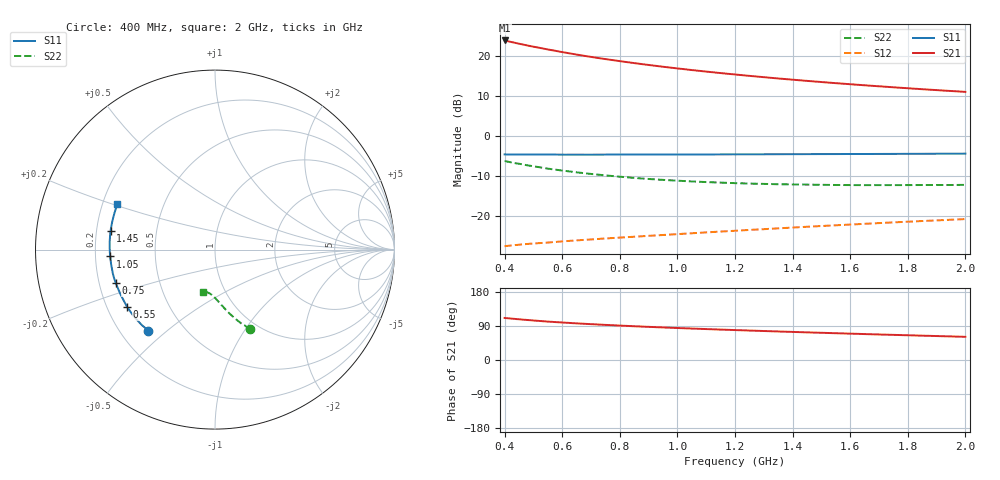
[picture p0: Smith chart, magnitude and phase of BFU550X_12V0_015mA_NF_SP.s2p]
! Filename:  P:\Prog\Test\Noise\ATS_data\Testdata_Net\BFU550X attenuator noise\BFU550X_APG2013_44_C05_12p0V_015mA_NF_CM01_D.sf
! Date/Time: Fri 26/Jul/2013 14:34:25
! BFU550X_APG2013_44_C05_12p0V_1to35mA_NF_CM01_Bias6_R.sf
! Noise Parameter Data File
! BFU550X_APG2013_44_C05_12p0V_1to35mA_NF_CM01
! Date/time: Mon Jul 22 11:28:10 2013
! VAR V_out= 12.001000
! VAR I_out= 14.995000
! VAR V_in= 0.783400
! VAR I_in= 0.144350
! Device data file deembeded for feedlines and parallel
! Original file: \BFU550X attenuator noise\BFU550X_APG2013_44_C05_12p0V_015mA_NF_CM01_R.sf
! Feed-files: PR005V01_100713_Feed1.s2p, PR005V01_100713_Feed2.s2p
! Parallel-file: PR005V01_100713_Par.s2p
# MHz S MA R 50
!  Freq-MHz  S11-mag  S11-arg  S21-mag  S21-arg  S12-mag  S12-arg  S22-mag  S22-arg
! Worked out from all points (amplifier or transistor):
!   37 points, 400 MHz to 2 GHz, reference 50 ohm
!   highest |S21| = 23.9 dB at 400 MHz (marker M1)
!   |S21| within 3 dB of that: start of sweep to 606.9 MHz
!   unconditionally stable (mu >= 1): 1.771 GHz to end of sweep
!   at 500 MHz: K = 0.51, MSG = 24.7 dB, |S12| = -27.0 dB
!   at 1.1 GHz: K = 0.85, MSG = 20.2 dB, |S12| = -24.2 dB
!   at 2 GHz: K = 1.03, MAG = 14.9 dB, |S12| = -20.8 dB
!   lowest NFmin = 0.94 dB at 460 MHz
!   S11 on the Smith chart (normalised r, x): 400 MHz: 0.31, -0.43; 550 MHz: 0.28, -0.28; 750 MHz: 0.27, -0.15; 1.05 GHz: 0.26, -0.03; 1.45 GHz: 0.26, +0.08; 2 GHz: 0.26, +0.21
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400  0.5867 -129.6  15.71 110.9  0.04152 44.7  0.4844 -66.1
420  0.5844 -132.1  15.11 109.5  0.04224 44.5  0.4679 -67.6
440  0.5854 -134.7  14.58 108.1  0.04297 44.1  0.4533 -68.7
460  0.5851 -137.1  14.06 106.8  0.04367 43.8  0.4418 -70.0
500  0.5853 -141.5  13.13 104.3  0.04487 43.4  0.4169 -72.2
550  0.5846 -146.8  12.13 101.4  0.04606 43.2  0.3888 -74.8
600  0.5824 -150.8  11.23 98.9  0.04765 43.4  0.3682 -76.9
650  0.5826 -154.8  10.45 96.7  0.04906 43.4  0.3497 -78.8
700  0.5824 -158.1  9.777 94.6  0.0504 43.7  0.3338 -80.5
750  0.5833 -161.3  9.177 92.7  0.05186 44.0  0.3202 -82.1
800  0.5843 -164.3  8.652 90.8  0.05316 44.3  0.3081 -83.7
850  0.5846 -167.1  8.176 89.1  0.0545 44.7  0.2975 -85.1
950  0.5845 -171.9  7.362 85.9  0.05733 45.6  0.2811 -87.7
1050  0.585 -176.2  6.69 83.0  0.06026 46.4  0.2688 -90.0
1100  0.586 -178.2  6.398 81.6  0.0618 46.8  0.2639 -91.0
1200  0.5873 178.0  5.884 79.0  0.06479 47.5  0.256 -93.0
1300  0.5886 174.6  5.444 76.5  0.06779 48.2  0.2504 -95.0
1450  0.591 169.7  4.894 72.9  0.07269 49.0  0.2453 -97.6
1500  0.5918 168.2  4.734 71.8  0.07423 49.2  0.2439 -98.4
1600  0.5932 165.2  4.443 69.5  0.07742 49.6  0.242 -100.0
1750  0.595 161.2  4.067 66.3  0.08244 50.0  0.2418 -102.5
2000  0.5998 154.9  3.562 61.2  0.09072 50.5  0.2435 -106.1
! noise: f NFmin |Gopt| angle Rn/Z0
400  1  0.1442  175.6  0.0918
460  0.942  0.1941  178.4  0.0753
600  0.9609  0.1826  177.1  0.0827
800  0.9727  0.2287  177.7  0.0719
1000  1.031  0.2515  -178.3  0.0671
1200  1.052  0.2641  -177  0.0694
1400  1.096  0.2967  -174.6  0.0621
1600  1.156  0.2901  -165.9  0.0756
1800  1.124  0.3194  -170.5  0.0643
2000  1.172  0.3328  -165.4  0.0731
